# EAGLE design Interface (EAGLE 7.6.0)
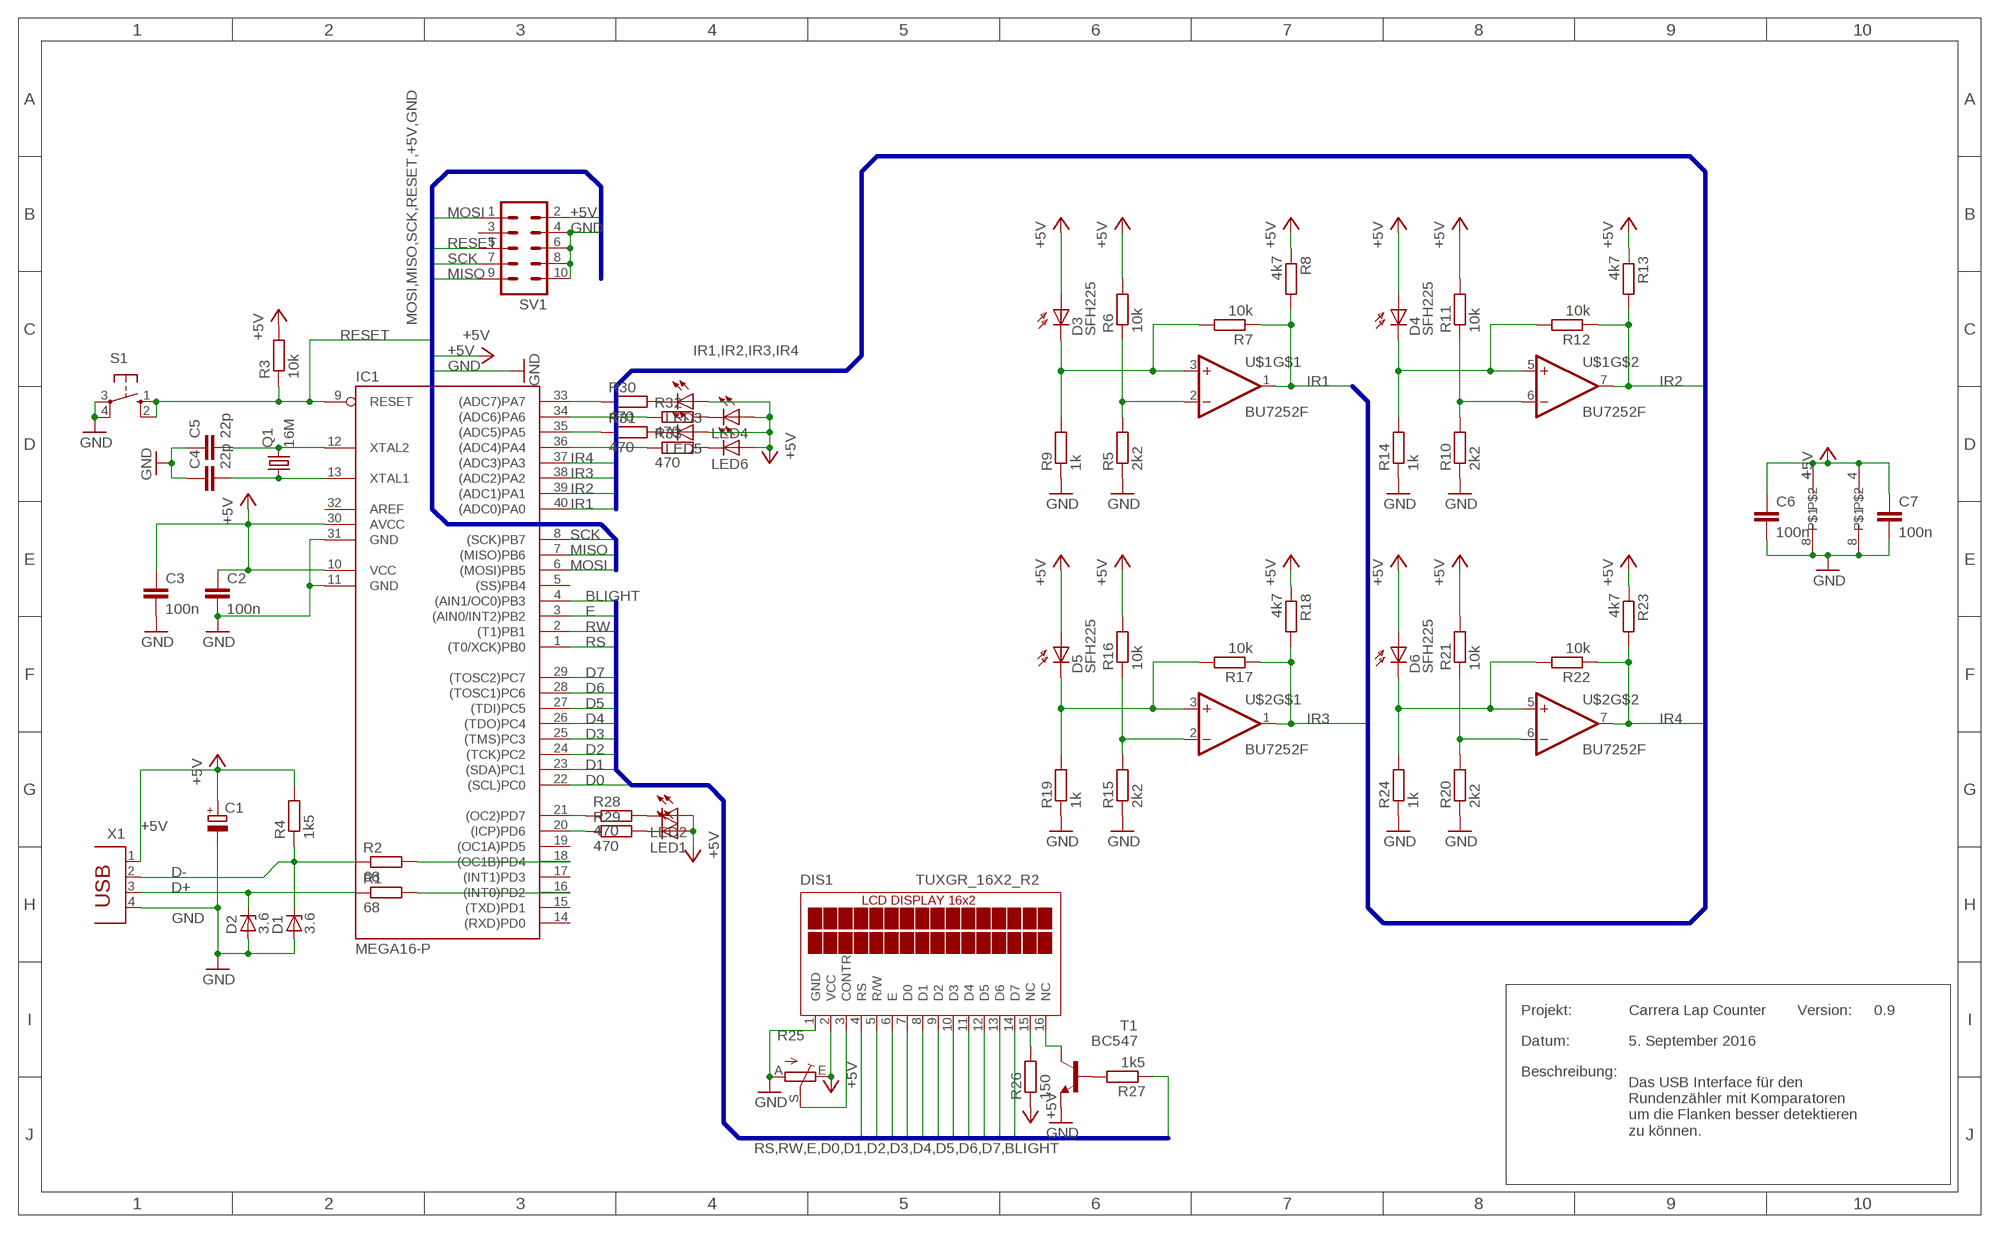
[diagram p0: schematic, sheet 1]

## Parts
C1  CPOL-EUE2.5-6  [E2,5-6]
C2  100n  C-EUC0805K  [C0805K]
C3  100n  C-EUC0805K  [C0805K]
C4  22p  C-EUC0805K  [C0805K]
C5  22p  C-EUC0805K  [C0805K]
C6  100n  C-EUC0805K  [C0805K]
C7  100n  C-EUC0805K  [C0805K]
D1  3.6  ZENER-DIODEZD-7.5  [ZDIO-7.5]
D2  3.6  ZENER-DIODEZD-7.5  [ZDIO-7.5]
D3  SFH225  [SFH225]
D4  SFH225  [SFH225]
D5  SFH225  [SFH225]
D6  SFH225  [SFH225]
DIS1  TUXGR_16X2_R2  [TUXGR_16X2_R2]
IC1  MEGA16-P  [DIL40]
LED1  LED5MM  [LED5MM]
LED2  LED5MM  [LED5MM]
LED3  LED5MM  [LED5MM]
LED4  LED5MM  [LED5MM]
LED5  LED5MM  [LED5MM]
LED6  LED5MM  [LED5MM]
Q1  16M  CRYSTALHC49S  [HC49/S]
R1  68  R-EU_R1210  [R1210]
R2  68  R-EU_R1210  [R1210]
R3  10k  R-EU_R1210  [R1210]
R4  1k5  R-EU_R1210  [R1210]
R5  2k2  R-EU_R1210  [R1210]
R6  10k  R-EU_R1210  [R1210]
R7  10k  R-EU_R1210  [R1210]
R8  4k7  R-EU_R1210  [R1210]
R9  1k  R-EU_R1210  [R1210]
R10  2k2  R-EU_R1210  [R1210]
R11  10k  R-EU_R1210  [R1210]
R12  10k  R-EU_R1210  [R1210]
R13  4k7  R-EU_R1210  [R1210]
R14  1k  R-EU_R1210  [R1210]
R15  2k2  R-EU_R1210  [R1210]
R16  10k  R-EU_R1210  [R1210]
R17  10k  R-EU_R1210  [R1210]
R18  4k7  R-EU_R1210  [R1210]
R19  1k  R-EU_R1210  [R1210]
R20  2k2  R-EU_R1210  [R1210]
R21  10k  R-EU_R1210  [R1210]
R22  10k  R-EU_R1210  [R1210]
R23  4k7  R-EU_R1210  [R1210]
R24  1k  R-EU_R1210  [R1210]
R25  TRIM_EU-LI10  [LI10]
R26  150  R-EU_R1210  [R1210]
R27  1k5  R-EU_R1210  [R1210]
R28  470  R-EU_R1210  [R1210]
R29  470  R-EU_R1210  [R1210]
R30  470  R-EU_R1210  [R1210]
R31  470  R-EU_R1210  [R1210]
R32  470  R-EU_R1210  [R1210]
R33  470  R-EU_R1210  [R1210]
S1  10-XX  [B3F-10XX]
SV1  MA05-2  [MA05-2]
T1  BC547  [TO92]
U$1  BU7252F  [SOP08]
U$2  BU7252F  [SOP08]
X1  PN61729  [PN61729]

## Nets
+5V: C1.+ C2.1 C3.1 C6.1 C7.1 D3.A D4.A D5.A D6.A DIS1.2(VCC) IC1.10(VCC) IC1.30(AVCC) LED1.A LED2.A LED3.A LED4.A LED5.A LED6.A R3.2 R4.2 R6.2 R8.1 R11.2 R13.1 R16.2 R18.1 R21.2 R23.1 R25.E R26.1 SV1.2 U$1.4 U$2.4 X1.1
BLIGHT: IC1.4((AIN1/OC0)PB3) R27.1
D0: DIS1.7(D0) IC1.22((SCL)PC0)
D1: DIS1.8(D1) IC1.23((SDA)PC1)
D2: DIS1.9(D2) IC1.24((TCK)PC2)
D3: DIS1.10(D3) IC1.25((TMS)PC3)
D4: DIS1.11(D4) IC1.26((TDO)PC4)
D5: DIS1.12(D5) IC1.27((TDI)PC5)
D6: DIS1.13(D6) IC1.28((TOSC1)PC6)
D7: DIS1.14(D7) IC1.29((TOSC2)PC7)
D+: D2.C R1.1 X1.3
D-: D1.C R2.1 R4.1 X1.2
E: DIS1.6(E) IC1.3((AIN0/INT2)PB2)
GND: C1.- C2.2 C3.2 C4.1 C5.1 C6.2 C7.2 D1.A D2.A DIS1.1(GND) IC1.11(GND) IC1.31(GND) R5.1 R9.1 R10.1 R14.1 R15.1 R19.1 R20.1 R24.1 R25.A S1.3(P) S1.4(P1) SV1.4 SV1.6 SV1.8 SV1.10 T1.1(E) U$1.8 U$2.8 X1.4
IR1: IC1.40((ADC0)PA0) R7.1 R8.2 U$1.1(OUT)
IR2: IC1.39((ADC1)PA1) R12.1 R13.2 U$1.7(OUT)
IR3: IC1.38((ADC2)PA2) R17.1 R18.2 U$2.1(OUT)
IR4: IC1.37((ADC3)PA3) R22.1 R23.2 U$2.7(OUT)
MISO: IC1.7((MISO)PB6) SV1.9
MOSI: IC1.6((MOSI)PB5) SV1.1
N$1: R10.2 R11.1 U$1.6(-IN)
N$2: R5.2 R6.1 U$1.2(-IN)
N$3: DIS1.3(CONTR) R25.S
N$4: D3.K(C) R7.2 R9.2 U$1.3(+IN)
N$5: IC1.16((INT0)PD2) R1.2
N$6: IC1.18((OC1B)PD4) R2.2
N$7: DIS1.16(NC) T1.3(C)
N$8: D4.K(C) R12.2 R14.2 U$1.5(+IN)
N$9: C5.2 IC1.12(XTAL2) Q1.2
N$10: C4.2 IC1.13(XTAL1) Q1.1
N$11: R15.2 R16.1 U$2.2(-IN)
N$12: DIS1.15(NC) R26.2
N$13: D5.K(C) R17.2 R19.2 U$2.3(+IN)
N$14: R20.2 R21.1 U$2.6(-IN)
N$15: R27.2 T1.2(B)
N$16: D6.K(C) R22.2 R24.2 U$2.5(+IN)
N$17: LED2.K(C) R28.2
N$18: LED1.K(C) R29.2
N$19: LED3.K(C) R30.2
N$20: LED5.K(C) R31.2
N$21: LED4.K(C) R32.2
N$22: LED6.K(C) R33.2
N$23: IC1.33((ADC7)PA7) R30.1
N$24: IC1.34((ADC6)PA6) R32.1
N$25: IC1.35((ADC5)PA5) R31.1
N$26: IC1.36((ADC4)PA4) R33.1
N$28: IC1.20((ICP)PD6) R29.1
N$29: IC1.21((OC2)PD7) R28.1
RESET: IC1.9(RESET) R3.1 S1.1(S) S1.2(S1) SV1.5
RS: DIS1.4(RS) IC1.1((T0/XCK)PB0)
RW: DIS1.5(R/W) IC1.2((T1)PB1)
SCK: IC1.8((SCK)PB7) SV1.7
Unconnected: IC1.5((SS)PB4) IC1.14((RXD)PD0) IC1.15((TXD)PD1) IC1.17((INT1)PD3) IC1.19((OC1A)PD5) IC1.32(AREF) SV1.3

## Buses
MOSI,MISO,SCK,RESET,+5V,GND
IR1,IR2,IR3,IR4
RS,RW,E,D0,D1,D2,D3,D4,D5,D6,D7,BLIGHT

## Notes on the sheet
- Projekt: | Carrera Lap Counter | Version: | 0.9
- Datum: | 5. September 2016
- Beschreibung:
- Das USB Interface für den
  Rundenzähler mit Komparatoren
  um die Flanken besser detektieren
  zu können.

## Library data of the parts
C1 = rcl:CPOL-EU: POLARIZED CAPACITOR, European symbol
C2-C7 = rcl:C-EU: CAPACITOR, European symbol
D1 D2 = diode:ZENER-DIODE: Z-Diode
D3-D6 = opto-trans-siemens:SFH225: PHOTO DIODE; OC_FARNELL: unknown; OC_NEWARK: unknown
DIS1 = display-lcd:TUXGR_16X2_R2: Tuxgraphics LCD display 16x2 characters reflective, without background light Source: tuxgr_12x2_r2.pdf; OC_FARNELL: unknown; OC_NEWARK: unknown
IC1 = atmel:MEGA16-P: MICROCONTROLLER 16 Kbytes FLASH 1 kbytes SRAM 512 bytes EEPROM USART 8-channel 10 bit ADC Source: avr.lbr; MPN: ATMEGA16-16PU; OC_FARNELL: 9171142; OC_NEWARK: 01M6885
LED1-LED6 = led:LED: LED
Q1 = crystal:CRYSTAL: CRYSTAL; OC_FARNELL: 1667008; OC_NEWARK: unknown
R1-R24 R26-R33 = rcl:R-EU_: RESISTOR, European symbol
R25 = pot:TRIM_EU-: POTENTIOMETER
S1 = switch-omron:10-XX: OMRON SWITCH; MPN: B3F-1000; OC_FARNELL: 176432; OC_NEWARK: 36M3542
SV1 = con-lstb:MA05-2: PIN HEADER; OC_FARNELL: unknown; OC_NEWARK: unknown
T1 = transistor-neu-to92:BC547: NPN TRANSISTOR
U$1 U$2 = RohmComparator:BU7252F
X1 = con-berg:PN61729: BERG USB connector; OC_FARNELL: unknown; OC_NEWARK: unknown

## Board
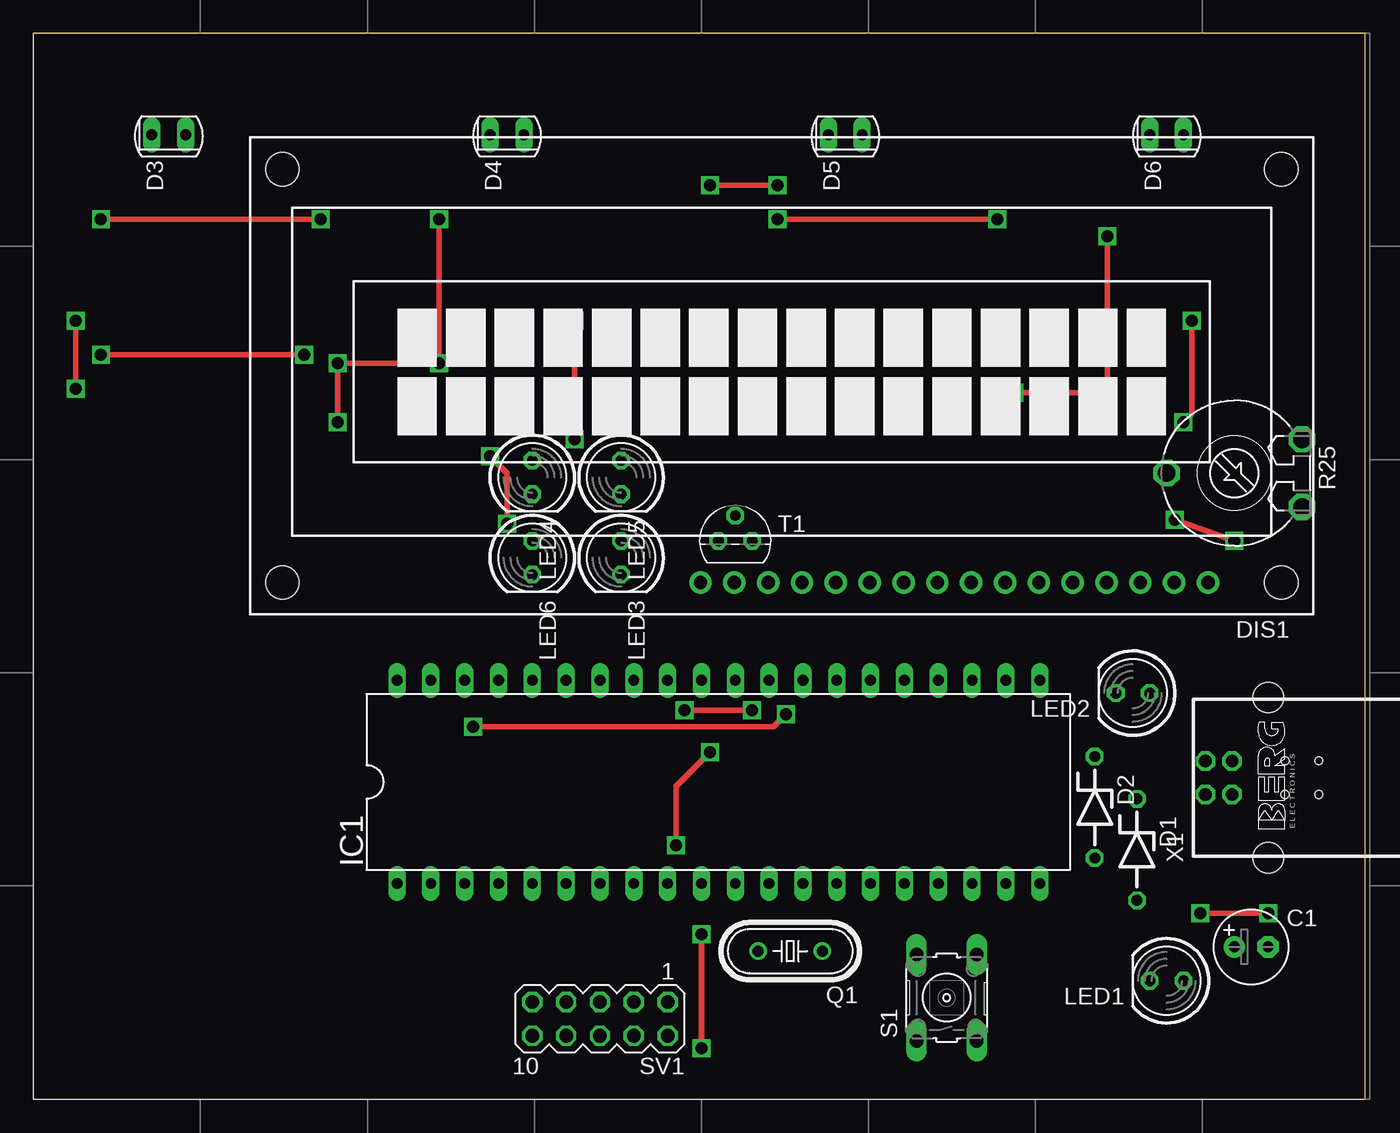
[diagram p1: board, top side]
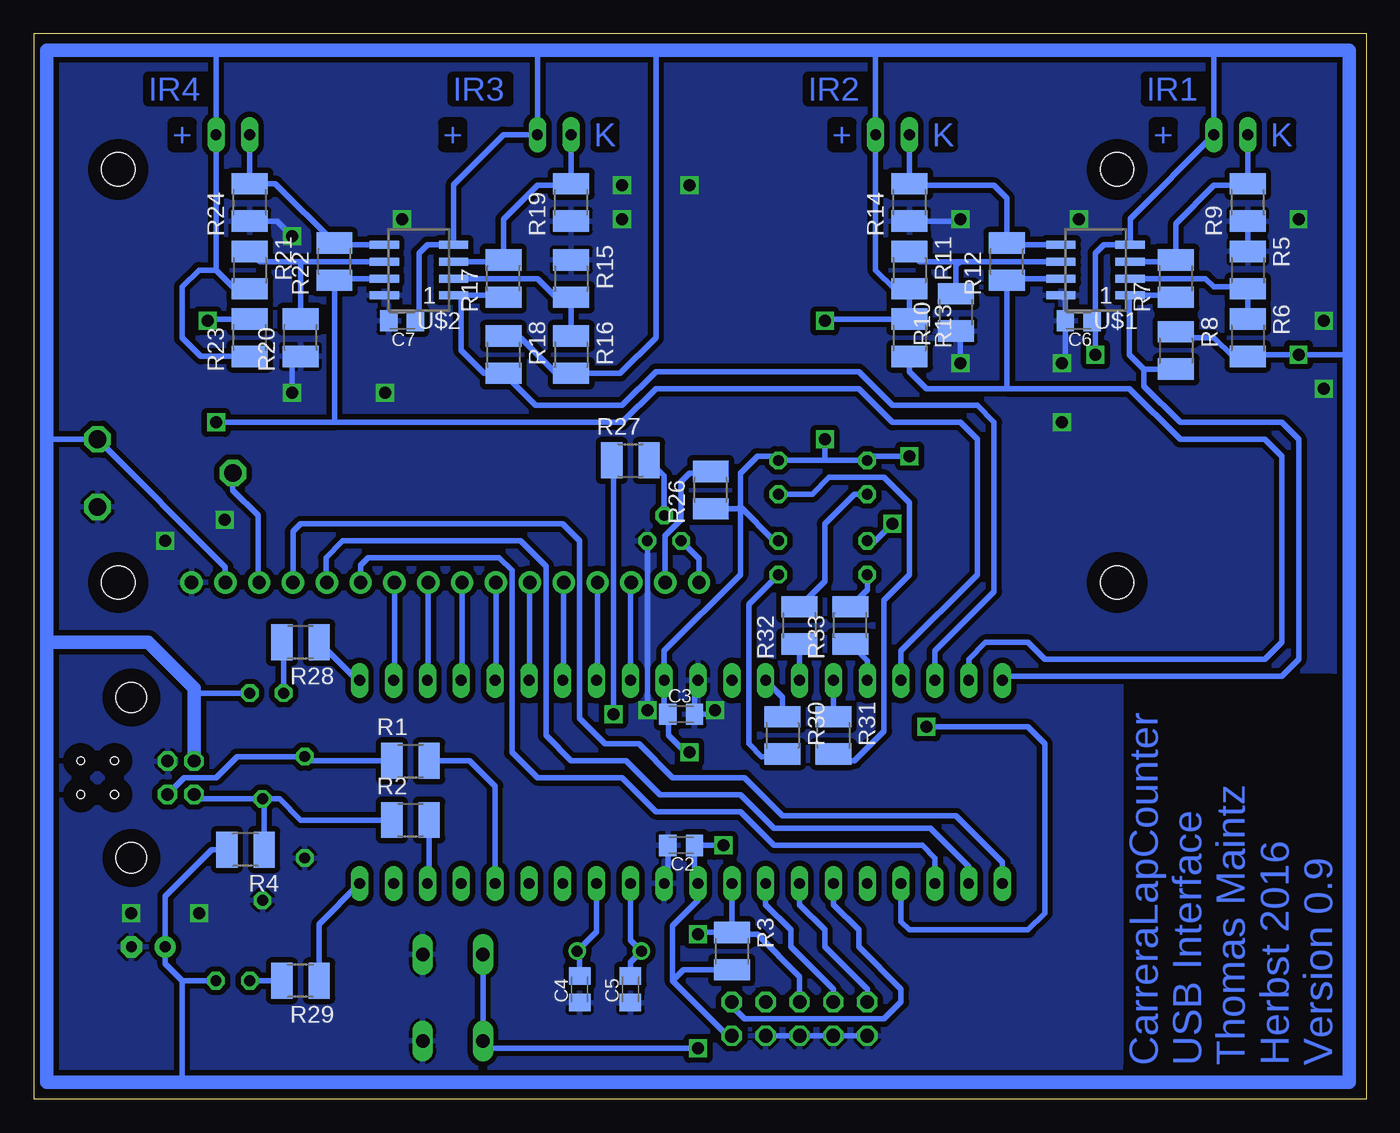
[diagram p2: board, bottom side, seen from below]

Size 100 x 80 mm. Coordinates in mm from the lower left corner, seen from the top.
Outline: 0,0 100,0 100,80 0,80 0,0
Copper layers (1*16): Top 0.035mm / dielectric 1.5mm / Bottom 0.035mm
Design rules "default *": minimum track width 10mil, minimum drill 24mil, track to track 0.02mm, track to pad 0.02mm, pad to pad 0.1mm, via to via 1mm, smd to smd 0.02mm, copper to edge 40mil, drill to drill 8mil, minimum pad ring 10mil, minimum via ring 8mil, stop-mask expansion 4mil, vias tented up to drill 0mil, thermal gap 10mil
Holes 0.6 mm at 93.98,25.4 93.98,22.86 96.52,25.4 96.52,22.86

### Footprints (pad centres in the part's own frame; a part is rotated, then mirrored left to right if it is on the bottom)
E2,5-6 = drill 0.813 pad 1.6: + -1.27,0 | drill 0.813 pad 1.6 octagon: - 1.27,0
C0805K = smd 1.3 x 1.6: 1 -1,0; 2 1,0
ZDIO-7.5 = drill 0.813 octagon: A 3.81,0; C -3.81,0
SFH225 = drill 0.813 long: A 0,1.27; K 0,-1.27
TUXGR_16X2_R2 = drill 1 pad 1.676: 1 -32,15.5; 2 -29.46,15.5; 3 -26.92,15.5; 4 -24.38,15.5; 5 -21.84,15.5; 6 -19.3,15.5; 7 -16.76,15.5; 8 -14.22,15.5; 9 -11.68,15.5; 10 -9.14,15.5; 11 -6.6,15.5; 12 -4.06,15.5; 13 -1.52,15.5; 14 1.02,15.5; 15 3.56,15.5; 16 6.1,15.5 | hole 2.5: -37.5,-15.5; 37.5,-15.5; -37.5,15.5; 37.5,15.5
DIL40 = drill 0.813 long: 1 -24.13,-7.62; 2 -21.59,-7.62; 3 -19.05,-7.62; 4 -16.51,-7.62; 5 -13.97,-7.62; 6 -11.43,-7.62; 7 -8.89,-7.62; 8 -6.35,-7.62; 9 -3.81,-7.62; 10 -1.27,-7.62; 11 1.27,-7.62; 12 3.81,-7.62; 13 6.35,-7.62; 14 8.89,-7.62; 15 11.43,-7.62; 16 13.97,-7.62; 17 16.51,-7.62; 18 19.05,-7.62; 19 21.59,-7.62; 20 24.13,-7.62; 21 24.13,7.62; 22 21.59,7.62; 23 19.05,7.62; 24 16.51,7.62; 25 13.97,7.62; 26 11.43,7.62; 27 8.89,7.62; 28 6.35,7.62; 29 3.81,7.62; 30 1.27,7.62; 31 -1.27,7.62; 32 -3.81,7.62; 33 -6.35,7.62; 34 -8.89,7.62; 35 -11.43,7.62; 36 -13.97,7.62; 37 -16.51,7.62; 38 -19.05,7.62; 39 -21.59,7.62; 40 -24.13,7.62
LED5MM = drill 0.813 octagon: A -1.27,0; K 1.27,0
HC49/S = drill 0.813: 1 -2.413,0; 2 2.413,0
R1210 = smd 1.6 x 2.7: 1 -1.4,0; 2 1.4,0
LI10 = drill 1.321 octagon: A -2.54,-5.08; E 2.54,-5.08; S 0,5.08
B3F-10XX = drill 1.016 long: 1 -3.251,2.261; 2 3.251,2.261; 3 -3.251,-2.261; 4 3.251,-2.261
MA05-2 = drill 1.016 octagon: 1 -5.08,-1.27; 2 -5.08,1.27; 3 -2.54,-1.27; 4 -2.54,1.27; 5 0,-1.27; 6 0,1.27; 7 2.54,-1.27; 8 2.54,1.27; 9 5.08,-1.27; 10 5.08,1.27
TO92 = drill 0.813 octagon: 1 1.27,0; 2 0,1.905; 3 -1.27,0
SOP08 = smd 0.6 x 2.2: 1 -1.905,-2.6; 2 -0.635,-2.6; 3 0.635,-2.6; 4 1.905,-2.6; 5 1.905,2.6; 6 0.635,2.6; 7 -0.635,2.6; 8 -1.905,2.6
PN61729 = drill 0.95 octagon: 1 1.25,4.71; 2 -1.25,4.71; 3 -1.25,2.71; 4 1.25,2.71 | hole 2.3: -6.02,0; 6.02,0

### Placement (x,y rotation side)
C1  91.44,11.43 0 top
C2  51.44,19.05 180 bottom
C3  51.44,28.89 0 bottom
C4  59.05,8.26 90 bottom
C5  55.24,8.26 90 bottom
C6  21.59,58.42 180 bottom
C7  72.39,58.42 180 bottom
D1  82.87,18.73 270 top
D2  79.69,21.91 270 top
D3  10.16,72.39 270 top
D4  35.56,72.39 270 top
D5  60.96,72.39 270 top
D6  85.09,72.39 270 top
DIS1  56.2,54.29 180 top
IC1  51.44,23.81 0 top
LED1  85.09,8.89 180 top
LED2  82.55,30.48 180 top
LED3  44.13,40.64 270 top
LED4  37.47,46.67 270 top
LED5  44.13,46.67 270 top
LED6  37.47,40.64 270 top
Q1  56.83,11.11 180 top
R1  71.75,25.4 0 bottom
R2  71.75,20.95 0 bottom
R3  47.62,11.11 270 bottom
R4  84.14,18.73 180 bottom
R5  8.89,62.23 270 bottom
R6  8.89,57.15 270 bottom
R7  14.29,61.59 90 bottom
R8  14.29,56.2 270 bottom
R9  8.89,67.31 90 bottom
R10  30.8,59.05 90 bottom
R11  34.29,62.23 270 bottom
R12  26.99,62.87 90 bottom
R13  34.29,57.15 270 bottom
R14  34.29,67.31 90 bottom
R15  59.69,61.59 270 bottom
R16  59.69,55.88 270 bottom
R17  64.77,61.59 90 bottom
R18  64.77,55.88 270 bottom
R19  59.69,67.31 90 bottom
R20  80.01,57.15 90 bottom
R21  83.82,62.23 270 bottom
R22  77.47,62.87 90 bottom
R23  83.82,57.15 90 bottom
R24  83.82,67.31 90 bottom
R25  90.17,46.99 90 top
R26  49.21,45.72 90 bottom
R27  55.24,47.94 0 bottom
R28  80.01,34.29 180 bottom
R29  80.01,8.89 180 bottom
R30  43.81,27.3 270 bottom
R31  40.01,27.3 270 bottom
R32  42.55,35.56 90 bottom
R33  38.73,35.56 90 bottom
S1  68.58,7.62 90 top
SV1  42.55,6.03 180 top
T1  52.7,41.91 0 top
U$1  20.32,62.23 90 bottom
U$2  71.12,62.23 90 bottom
X1  92.71,24.13 90 top

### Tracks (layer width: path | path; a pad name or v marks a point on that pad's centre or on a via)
+5V  (via drill 0.9)
  Top 0.406: v48.26,19.05 48.26,23.5 v50.8,26.04 | v20.32,55.88 v5.08,55.88 | v35.56,43.18 35.56,46.99 v34.29,48.26 | v40.64,58.42 v40.64,49.53
  Bottom 0.406: 20.32,58.69 20.32,63.5 19.68,64.14 U$1.4 17.72,66.1 D3.A 11.43,78.74 | 20.32,58.69 C6.1 | R4.2 86.68,18.73 90.17,15.24 C1.+ 90.17,10.16 88.9,8.89 | LED1.A 88.9,8.89 | 88.9,1.27 88.9,8.89 | LED2.A 88,30.48 | 99.06,49.53 R25.E 85.66,39.94 DIS1.2 | LED3.A 44.45,41.91 46.99,44.45 | 46.99,44.45 46.99,46.99 45.72,48.26 44.45,48.26 LED5.A 40.64,47.94 | 40.64,47.94 LED4.A 37.15,48.26 v34.29,48.26 | v48.26,19.05 C2.1 50.44,16.46 IC1.10 50.16,14.92 52.07,13.02 52.07,8.89 | v50.8,26.04 51.12,26.04 52.39,27.3 52.39,28.84 C3.1 52.7,29.16 IC1.30 52.7,33.66 46.99,39.37 46.99,44.45 | R8.1 13.84,57.15 11.43,57.15 10.03,55.75 R6.2 8.76,55.88 v5.08,55.88 1.27,55.88 | 36.83,78.74 D4.A 36.83,62.23 35.43,60.83 R11.2 R13.1 40.51,58.55 v40.64,58.42 | 20.32,58.69 v20.32,55.88 | R18.1 64.64,57.15 63.5,57.15 60.83,54.48 R16.2 56.01,54.48 53.34,57.15 53.34,78.74 | C7.1 71.12,58.69 71.12,63.5 70.48,64.14 U$2.4 68.52,68.64 64.77,72.39 D5.A 62.23,78.74 | R21.2 84.96,60.83 86.36,62.23 | 86.36,62.23 D6.A 86.36,78.74 | R23.1 87.5,55.75 88.9,57.15 88.9,60.96 87.63,62.23 86.36,62.23 | LED6.A 36.83,41.91 v35.56,43.18 | R26.1 47.12,44.32 46.99,44.45 | v40.64,49.53 40.64,47.94 | SV1.2 47.94,4.76 52.07,8.89 | R3.2 51.25,9.71 52.07,8.89
  Bottom 1.016: X1.1 88,30.48 88,30.85 91.44,34.29 99.06,34.29 | 99.06,34.29 99.06,49.53 99.06,78.74 86.36,78.74 62.23,78.74 53.34,78.74 36.83,78.74 11.43,78.74 1.27,78.74 1.27,55.88 1.27,1.27 88.9,1.27 99.06,1.27 99.06,34.29
BLIGHT  (via drill 0.9)
  Top 0.406: v33.02,27.94 55.56,27.94 v56.52,28.89
  Bottom 0.406: IC1.4 34.92,13.34 34.29,12.7 25.4,12.7 24.13,13.97 24.13,26.67 25.4,27.94 v33.02,27.94 | v56.52,28.89 56.52,47.81 R27.1
D0
  Bottom 0.406: DIS1.7 72.96,31.5 IC1.22
D1
  Bottom 0.406: DIS1.8 70.42,31.5 IC1.23
D2
  Bottom 0.406: DIS1.9 67.88,31.5 IC1.24
D3
  Bottom 0.406: DIS1.10 65.34,31.5 IC1.25
D4
  Bottom 0.406: DIS1.11 62.8,31.5 IC1.26
D5
  Bottom 0.406: DIS1.12 60.26,31.5 IC1.27
D6
  Bottom 0.406: DIS1.13 57.72,31.5 IC1.28
D7
  Bottom 0.406: IC1.29 55.24,38.73 DIS1.14
D+
  Bottom 0.406: R1.1 79.38,25.4 D2.C 84.77,25.72 86.36,24.13 88.75,24.13 X1.3
D-
  Bottom 0.406: R2.1 80.01,20.95 81.6,22.54 D1.C | R4.1 82.74,22.41 D1.C | D1.C 87.66,22.54 X1.2
E
  Bottom 0.406: DIS1.6 75.5,40.07 74.93,40.64 65.09,40.64 64.14,39.69 64.14,26.04 62.23,24.13 55.88,24.13 53.34,21.59 46.99,21.59 44.45,19.05 33.34,19.05 32.38,18.1 IC1.3
GND  (via drill 0.9)
  Top 0.406: v30.48,66.04 v30.48,55.24 v22.86,55.24 v22.86,50.8 | v5.08,66.04 v21.59,66.04 | v80.64,64.77 v80.64,53.02 v73.66,53.02 | v55.88,66.04 v72.39,66.04 | v48.9,29.21 v53.98,29.21 | v90.17,41.91 v85.72,43.5 | v92.71,13.97 v87.63,13.97 | v3.17,53.34 v3.17,58.42 | v55.88,68.58 v50.8,68.58
  Bottom 0.406: R9.1 R5.1 | U$1.8 22.59,59.99 C6.2 22.59,55.52 v22.86,55.24 | C2.2 52.44,16.46 IC1.11 | IC1.31 50.44,31.16 C3.2 49.21,28.89 v48.9,29.21 | SV1.10 SV1.8 SV1.6 SV1.4 | R14.1 30.61,65.91 v30.48,66.04 | v30.48,55.24 30.48,57.34 R10.1 | R24.1 81.78,65.91 v80.64,64.77 | v80.64,53.02 80.64,55.12 R20.1 | v53.98,29.21 T1.1
  pour Bottom (isolate 0.406): 0,80.01 100.33,80.01 100.33,0 0,0
IR1
  Bottom 0.406: R7.1 14.42,60.33 U$1.1 17.78,60.27 17.78,55.88 16.7,54.8 | R8.2 16.7,54.8 | 16.7,54.8 16.7,53.53 13.97,50.8 6.35,50.8 5.08,49.53 5.08,33.02 6.35,31.75 26.99,31.75 IC1.40
IR2
  Bottom 0.406: U$1.7 26.86,61.59 R12.1 26.99,53.34 | 26.99,53.34 33.02,53.34 34.29,54.61 R13.2 | 26.99,53.34 17.78,53.34 13.97,49.53 7.62,49.53 6.35,48.26 6.35,34.29 7.62,33.02 24.13,33.02 25.4,34.29 28.57,34.29 29.84,33.02 IC1.39
IR3
  Bottom 0.406: U$2.1 67.94,60.33 | 67.94,60.33 64.9,60.33 R17.1 | 67.94,60.33 67.94,56.2 66.23,54.48 R18.2 62.36,52.07 55.88,52.07 53.34,54.61 38.1,54.61 35.56,52.07 29.21,52.07 27.94,50.8 27.94,38.1 32.38,33.66 IC1.38
IR4  (via drill 0.9)
  Top 0.406: v87,58.42 87,51.44 v86.36,50.8
  Bottom 0.406: U$2.7 77.34,61.59 R22.1 77.47,50.8 | R23.2 86.86,58.55 v87,58.42 | v86.36,50.8 77.47,50.8 | IC1.37 34.92,33.66 29.21,39.37 29.21,49.53 30.48,50.8 35.56,50.8 38.1,53.34 53.34,53.34 55.88,50.8 77.47,50.8
MISO
  Bottom 0.406: SV1.9 37.47,8.26 40.64,11.43 40.64,12.7 42.55,14.61 IC1.7
MOSI
  Bottom 0.406: SV1.1 47.62,6.99 46.67,6.03 36.2,6.03 34.92,7.3 34.92,8.26 38.1,11.43 38.1,12.7 40.01,14.61 IC1.6
N$1
  Bottom 0.406: U$1.6 30.48,62.87 | 30.48,62.87 33.52,62.87 R11.1 33.66,62.99 | R10.2 30.8,62.55 30.48,62.87
N$2
  Bottom 0.406: R6.1 R5.2 9.02,60.96 11.43,60.96 12.06,61.59 U$1.2
N$3
  Bottom 0.406: R25.S 85.09,45.72 83.19,43.81 83.19,38.86 DIS1.3
N$4
  Bottom 0.406: D3.K R9.2 9.02,68.58 11.43,68.58 14.29,65.72 R7.2 14.42,62.87 U$1.3
N$5
  Bottom 0.406: IC1.16 65.41,23.5 67.31,25.4 R1.2
N$6
  Bottom 0.406: R2.2 70.36,16.32 IC1.18
N$7
  Bottom 0.406: DIS1.16 50.1,40.57 T1.3
N$8
  Bottom 0.406: U$1.5 26.86,64.14 R12.2 26.99,67.63 27.94,68.58 34.16,68.58 R14.2 D4.K
N$9
  Bottom 0.406: IC1.12 55.24,11.94 Q1.2 55.24,10.29 C5.2
N$10
  Bottom 0.406: C4.2 59.05,10.92 Q1.1 57.78,12.57 IC1.13
N$11
  Bottom 0.406: U$2.2 62.23,61.59 60.96,60.33 59.82,60.33 R15.2 R16.1
N$12
  Bottom 0.406: DIS1.15 52.64,42.3 51.44,43.5 51.44,46.35 50.8,46.99 49.34,46.99 R26.2
N$13
  Bottom 0.406: U$2.3 64.9,62.87 R17.2 64.77,66.04 62.23,68.58 59.82,68.58 R19.2 D5.K
N$14
  Bottom 0.406: U$2.6 80.01,62.87 | 80.01,62.87 83.06,62.87 R21.1 | R20.2 80.01,62.87
N$15
  Bottom 0.406: T1.2 52.7,46.8 R27.2
N$16
  Bottom 0.406: U$2.5 77.34,64.14 R22.2 81.92,68.71 R24.2 D6.K
N$17
  Bottom 0.406: LED2.K 81.28,34.16 R28.2
N$18
  Bottom 0.406: R29.2 LED1.K
N$19
  Bottom 0.406: R30.2 45.27,25.72 45.4,25.72 46.35,26.67 46.35,37.15 LED3.K
N$20
  Bottom 0.406: LED5.K 41.59,45.4 40.32,46.67 36.2,46.67 34.29,44.77 34.29,39.37 36.2,37.47 36.2,27.62 38.42,25.4 39.5,25.4 R31.2
N$21
  Bottom 0.406: LED4.K 38.42,45.4 40.64,43.18 40.64,38.87 R32.2
N$22
  Bottom 0.406: LED6.K 37.47,38.23 R33.2
N$23
  Bottom 0.406: R30.1 43.81,30.16 IC1.33
N$24
  Bottom 0.406: R32.1 IC1.34
N$25
  Bottom 0.406: R31.1 IC1.35
N$26
  Bottom 0.406: IC1.36 37.47,32.89 R33.1
N$28
  Bottom 0.406: R29.1 78.61,13.15 IC1.20
N$29
  Bottom 0.406: IC1.21 75.75,31.43 R28.1
RESET  (via drill 0.9)
  Top 0.406: v50.16,12.38 v50.16,3.81
  Bottom 0.406: S1.2 S1.1 65.76,3.81 v50.16,3.81 | R3.1 50.03,12.51 v50.16,12.38 | R3.1 IC1.9 | SV1.5 42.55,9.21 45.72,12.38 47.49,12.38 R3.1
RS
  Bottom 0.406: DIS1.4 80.58,42.61 80.01,43.18 60.33,43.18 59.05,41.91 59.05,28.57 57.15,26.67 54.61,26.67 52.07,24.13 46.67,24.13 43.81,21.27 30.8,21.27 27.3,17.78 IC1.1
RW
  Bottom 0.406: DIS1.5 78.11,38.86 78.11,40.64 76.83,41.91 63.5,41.91 61.59,40.01 61.59,27.3 59.69,25.4 55.56,25.4 53.02,22.86 46.99,22.86 44.45,20.32 32.7,20.32 29.84,17.46 IC1.2
SCK
  Bottom 0.406: SV1.7 40.01,8.26 43.18,11.43 43.18,12.7 45.09,14.61 IC1.8

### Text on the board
Bottom: IR1 | IR2 | IR3 | IR4 | K | + | K | + | K | + | + | CarreraLapCounter / USB Interface / Thomas Maintz / Herbst 2016 / Version 0.9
